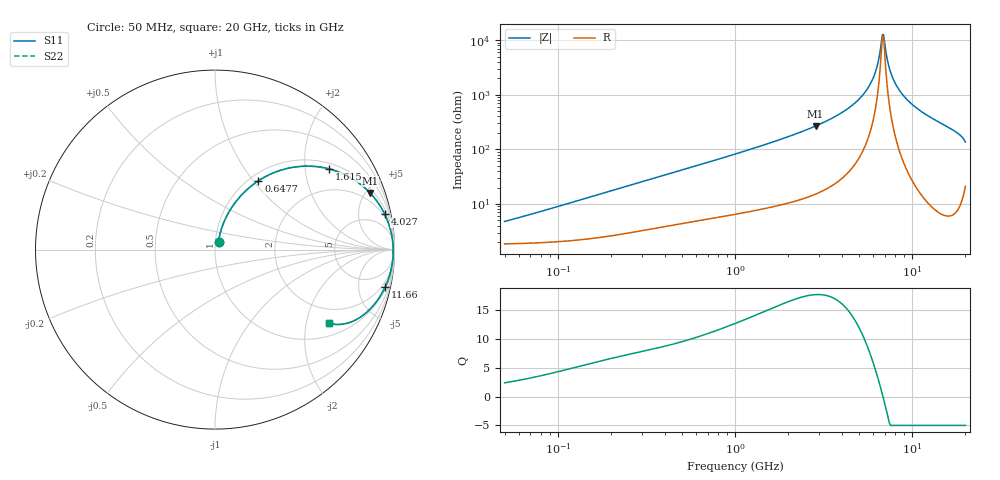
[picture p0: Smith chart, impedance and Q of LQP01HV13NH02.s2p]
!Murata Part Number: LQP01HV13NH02
!These Parameters are Measured in Series Mode Connection
!  o--[Z]--o
!Port1  Port2
!  o-------o
!Freq. Start=50[MHz] Stop=20[GHz], 401[Steps]
# Hz S RI R 50
!Freq.(Hz) S11(Real) S11(Imag) S21(Real) S21(Imag) S12(Real) S12(Imag) S22(Real) S22(Imag)
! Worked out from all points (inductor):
!   401 points, 50 MHz to 20 GHz, reference 50 ohm
!   read as one part in series: L = 14 nH near 65.47 MHz
!   highest Q = 17.6 at 2.853 GHz (marker M1), where L = 14.9 nH
!   self-resonance near 6.802 GHz
!   S11 on the Smith chart (normalised r, x): 50 MHz: 1.04, +0.09; 647.7 MHz: 1.10, +1.06; 1.615 GHz: 1.18, +2.68; 4.027 GHz: 1.59, +9.45; 11.66 GHz: 1.25, -9.16; 20 GHz: 1.42, -2.71
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5e7  0.0201 0.0424  0.9799 -0.0424  0.9799 -0.0424  0.0201 0.0424
1.364002e8  0.0348 0.1122  0.9652 -0.1122  0.9652 -0.1122  0.0348 0.1122
3.721004e8  0.1156 0.2661  0.8844 -0.2661  0.8844 -0.2661  0.1156 0.2661
6.476653e8  0.2416 0.3832  0.7584 -0.3832  0.7584 -0.3832  0.2416 0.3832
1e9  0.4076 0.4534  0.5924 -0.4534  0.5924 -0.4534  0.4076 0.4534
1.614971e9  0.6352 0.4497  0.3648 -0.4497  0.3648 -0.4497  0.6352 0.4497
2.728004e9  0.8497 0.3301  0.1503 -0.3301  0.1503 -0.3301  0.8497 0.3301
2.853386e9  0.8638 0.3158  0.1362 -0.3158  0.1362 -0.3158  0.8638 0.3158
4.026975e9  0.9461 0.1968  0.0539 -0.1968  0.0539 -0.1968  0.9461 0.1968
4.966507e9  0.9752 0.1199  0.0248 -0.1199  0.0248 -0.1199  0.9752 0.1199
5.769027e9  0.9872 0.0642  0.0128 -0.0642  0.0128 -0.0642  0.9872 0.0642
6.217679e9  0.9907 0.0362  0.00935 -0.0362  0.00935 -0.0362  0.9907 0.0362
6.406762e9  0.9916 0.025  0.00844 -0.025  0.00844 -0.025  0.9916 0.025
6.701223e9  0.9924 0.00813  0.00758 -0.00813  0.00758 -0.00813  0.9924 0.00813
6.802353e9  0.9926 0.00249  0.00743 -0.00249  0.00743 -0.00249  0.9926 0.00249
7.009217e9  0.9927 -0.0088  0.00733 0.0088  0.00733 0.0088  0.9927 -0.0088
7.442007e9  0.9921 -0.0315  0.00794 0.0315  0.00794 0.0315  0.9921 -0.0315
8.020766e9  0.9898 -0.0599  0.0102 0.0599  0.0102 0.0599  0.9898 -0.0599
8.774992e9  0.9846 -0.0944  0.0154 0.0944  0.0154 0.0944  0.9846 -0.0944
1.166392e10  0.9493 -0.2059  0.0507 0.2059  0.0507 0.2059  0.9493 -0.2059
1.696185e10  0.8308 -0.3613  0.1692 0.3613  0.1692 0.3613  0.8308 -0.3613
2e10  0.6327 -0.4107  0.3673 0.4107  0.3673 0.4107  0.6327 -0.4107
